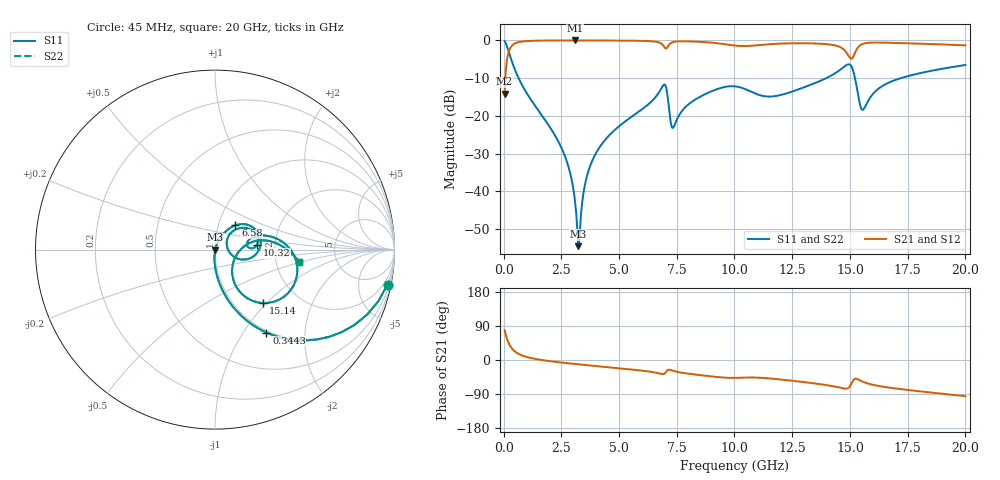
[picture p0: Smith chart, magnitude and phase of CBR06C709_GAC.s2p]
! S-parameter model data by Modelithics Inc.  support@modelithics.com 813-866-6335  Tampa FL USA
! S-Parameter data specifications:
! Substrate: 20-mil Rogers 4350B, substrate thickness, H=0.508mm, Dielectric constant, Er=3.75
! PCB Mounting Pad Footprint: Pad width, PadW=0.85mm , Pad length, PadL=0.64mm , Pad gap, PadG (edge-to-edge)=0.62mm , Reference planes=1.9mm apart
#  GHz  S  MA  R 50
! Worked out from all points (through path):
!   801 points, 45 MHz to 20 GHz, reference 50 ohm
!   highest |S21| = -0.02 dB at 3.088 GHz (marker M1); lowest = -14.2 dB at 45 MHz (marker M2)
!   group delay of S21, straight-line fit = 14.2 ps
!   lowest |S11| = -54.5 dB at 3.238 GHz (marker M3), VSWR 1.00, Z = 50.2 - j0.0897 ohm
!   |S11| at or under -10 dB: 650.1 MHz to 13.98 GHz (13.33 GHz wide, 182 % of centre); 15.22 GHz to 17.21 GHz (1.989 GHz wide, 12.3 % of centre)
!   |S22| runs from -54.5 to -0.2 dB; largest |S21 - S12| = 0
!   S11 on the Smith chart (normalised r, x): 45 MHz: 0.97, -9.88; 344.3 MHz: 0.97, -1.28; 6.58 GHz: 1.21, +0.34; 10.32 GHz: 1.61, +0.09; 15.14 GHz: 1.34, -0.95; 20 GHz: 2.70, -0.46
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0.045  0.9806 -11.5  0.1958 78.5  0.1958 78.5  0.9806 -11.5
0.344325  0.5433 -58.2  0.8389 31.7  0.8389 31.7  0.5433 -58.2
0.868144  0.2351 -79.2  0.971 10.5  0.971 10.5  0.2351 -79.2
2.514431  0.03723 -94.4  0.9976 -6.8  0.9976 -6.8  0.03723 -94.4
3.088138  0.007671 -87.4  0.9981 -10.5  0.9981 -10.5  0.007671 -87.4
3.2378  0.001875 -28.5  0.998 -11.4  0.998 -11.4  0.001875 -28.5
3.387462  0.00641 60.9  0.998 -12.3  0.998 -12.3  0.00641 60.9
3.661844  0.01804 69.8  0.9977 -14.0  0.9977 -14.0  0.01804 69.8
4.160719  0.03848 69.8  0.9968 -16.9  0.9968 -16.9  0.03848 69.8
6.580262  0.177 49.9  0.963 -33.2  0.963 -33.2  0.177 49.9
6.704981  0.1994 45.2  0.9458 -34.9  0.9458 -34.9  0.1994 45.2
7.004306  0.2552 5.4  0.7889 -33.9  0.7889 -33.9  0.2552 5.4
7.353519  0.07011 20.8  0.9528 -28.8  0.9528 -28.8  0.07011 20.8
8.276438  0.1625 43.9  0.9642 -38.2  0.9642 -38.2  0.1625 43.9
10.0225  0.246 12.8  0.8535 -47.2  0.8535 -47.2  0.246 12.8
10.32183  0.2348 6.4  0.8409 -46.7  0.8409 -46.7  0.2348 6.4
13.36496  0.2627 17.4  0.9124 -61.0  0.9124 -61.0  0.2627 17.4
14.83664  0.4684 -12.0  0.6991 -75.7  0.6991 -75.7  0.4684 -12.0
15.13597  0.3998 -48.2  0.6007 -54.3  0.6007 -54.3  0.3998 -48.2
15.56001  0.1206 -20.7  0.8998 -57.3  0.8998 -57.3  0.1206 -20.7
16.68248  0.2755 10.8  0.93 -72.7  0.93 -72.7  0.2755 10.8
20  0.4722 -8.1  0.859 -95.5  0.859 -95.5  0.4722 -8.1
